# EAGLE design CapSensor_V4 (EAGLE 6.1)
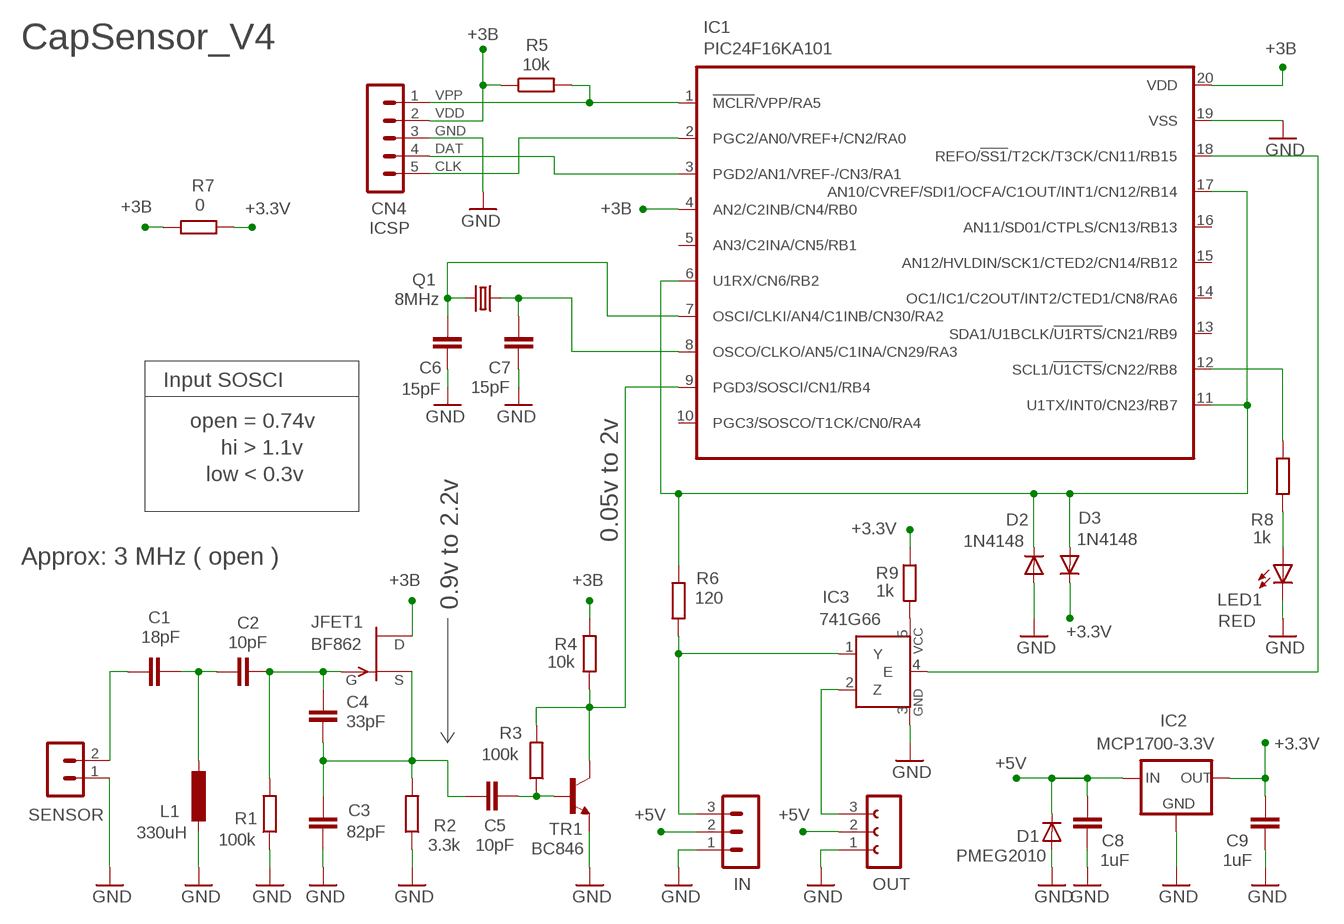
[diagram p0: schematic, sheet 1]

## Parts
C1  18pF  C-EUC0805  [C0805]
C2  10pF  C-EUC0805  [C0805]
C3  82pF  C-EUC0805  [C0805]
C4  33pF  C-EUC0805  [C0805]
C5  10pF  C-EUC0805  [C0805]
C6  15pF  C-EUC0603  [C0603]
C7  15pF  C-EUC0603  [C0603]
C8  1uF  C-EUC0603  [C0603]
C9  1uF  C-EUC0603  [C0603]
CN4  ICSP  MA05-1  [MA05-1]
D1  PMEG2010  DIODE-SOD123-B  [SOD123-B]
D2  1N4148  DIODE-SOD123-B  [SOD123-B]
D3  1N4148  DIODE-SOD123-B  [SOD123-B]
IC1  PIC24F16KA101  PIC24F04KA201SOIC  [SOIC20_S]
IC2  MCP1700-3.3V  MCP1700SOT23  [SOT23]
IC3  741G66  741G66SOT23-5L  [SOT23-5L]
IN  MA03-1N  [MA03-1]
JFET1  BF862  BF861NR  [SOT23]
L1  330uH  INDUCTORL1210  [L1210]
LED1  RED  LED3MM_F  [LED3MM]
OUT  FE03-1"  [FE03-1]
Q1  8MHz  CRYSTALC4  [CRYSTAL_4]
R1  100k  R-EU_R0805  [R0805]
R2  3.3k  R-EU_R0805  [R0805]
R3  100k  R-EU_R0805  [R0805]
R4  10k  R-EU_R0805  [R0805]
R5  10k  R-EU_R0805  [R0805]
R6  120  R-EU_R0805  [R0805]
R7  0  R-EU_R1206_L  [R1206_L]
R8  1k  R-EU_R0805_L  [R0805_L]
R9  1k  R-EU_R0603  [R0603]
SENSOR  Sensor  MA02-1N  [MA02-1]
TR1  BC846  BC846N  [SOT23]

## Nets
+3.3V: C9.1 D3.C IC2.2(OUT) R7.2 R9.1
+3B: CN4.2 IC1.4(AN2/C2INB/CN4/RB0) IC1.20(VDD) JFET1.2(D) R4.2 R5.1 R7.1
+5V: C8.1 D1.C IC2.3(IN) IN.2 OUT.2
GND: C3.1 C6.1 C7.1 C8.2 C9.2 CN4.3 D1.A D2.A IC1.19(VSS) IC2.1(GND) IC3.3(GND) IN.1 L1.2 LED1.K(C) OUT.1 R1.1 R2.1 SENSOR.1 TR1.2(E)
N$1: IC1.18(REFO/!SS1!/T2CK/T3CK/CN11/RB15) IC3.4(E)
N$2: IC1.9(PGD3/SOSCI/CN1/RB4) R3.2 R4.1 TR1.3(C)
N$3: D2.C D3.A IC1.6(U1RX/CN6/RB2) IC1.11(U1TX/INT0/CN23/RB7) IC1.17(AN10/CVREF/SDI1/OCFA/C1OUT/INT1/CN12/RB14) R6.1
N$4: C5.2 R3.1 TR1.1(B)
N$5: C1.2 C2.1 L1.1
N$6: LED1.A R8.2
N$7: C3.2 C4.1 C5.1 JFET1.1(S) R2.2
N$8: IC1.12(SCL1/!U1CTS!/CN22/RB8) R8.1
N$9: C2.2 C4.2 JFET1.3(G) R1.2
N$10: C1.1 SENSOR.2
N$11: IC3.5(VCC) R9.2
N$13: C6.2 IC1.7(OSCI/CLKI/AN4/C1INB/CN30/RA2) Q1.3
N$14: C7.2 IC1.8(OSCO/CLKO/AN5/C1INA/CN29/RA3) Q1.1
N$15: IC3.2(Z) OUT.3
N$16: IC3.1(Y) IN.3 R6.2
N$18: CN4.4 IC1.3(PGD2/AN1/VREF-/CN3/RA1)
N$19: CN4.1 IC1.1(!MCLR!/VPP/RA5) R5.2
N$20: CN4.5 IC1.2(PGC2/AN0/VREF+/CN2/RA0)
Unconnected: IC1.5(AN3/C2INA/CN5/RB1) IC1.10(PGC3/SOSCO/T1CK/CN0/RA4) IC1.13(SDA1/U1BCLK/!U1RTS!/CN21/RB9) IC1.14(OC1/IC1/C2OUT/INT2/CTED1/CN8/RA6) IC1.15(AN12/HVLDIN/SCK1/CTED2/CN14/RB12) IC1.16(AN11/SD01/CTPLS/CN13/RB13)

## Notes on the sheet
- CapSensor_V4
- Input SOSCI
- open = 0.74v
- hi > 1.1v
- low < 0.3v
- 0.05v to 2v
- Approx: 3 MHz ( open )
- 0.9v to 2.2v

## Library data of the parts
C1-C9 = 00-LIVIO:C-EU: CAPACITOR, European symbol
CN4 = 03-con-lstb-M:MA05-1: PIN HEADER; CLK: CLK; DAT: DAT; GND: GND; VDD: VDD; VPP: VPP
D1-D3 = 00-LIVIO:DIODE-: DIODE
IC1 = 00-LIVIO:PIC24F04KA201
IC2 = 00-LIVIO:MCP1700: Linear regulator Quescient courrent 1.8uA Input 2.3v to 6v Output 1.2v 1.8v 2.5v 3.0v 3.3v 5.0v
IC3 = 00-LIVIO:74*1G66: Single Analog / Bilateral Switch Source: http://www.semiconductors.philips.com/acrobat_download/datasheets/74HC_HCT1G66_3.pdf
IN = 03-con-lstb-M:MA03-1: PIN HEADER
JFET1 = 00-LIVIO:BF861
L1 = 00-LIVIO:INDUCTOR
LED1 = 00-LIVIO:LED: LEDS
OUT = 02-con-lsta-F:FE03-1: FEMALE HEADER
Q1 = 00-LIVIO:CRYSTAL: CRYSTAL
R1-R9 = 00-LIVIO:R-EU_: RESISTOR, European symbol
SENSOR = 03-con-lstb-M:MA02-1: PIN HEADER
TR1 = 00-LIVIO:BC846

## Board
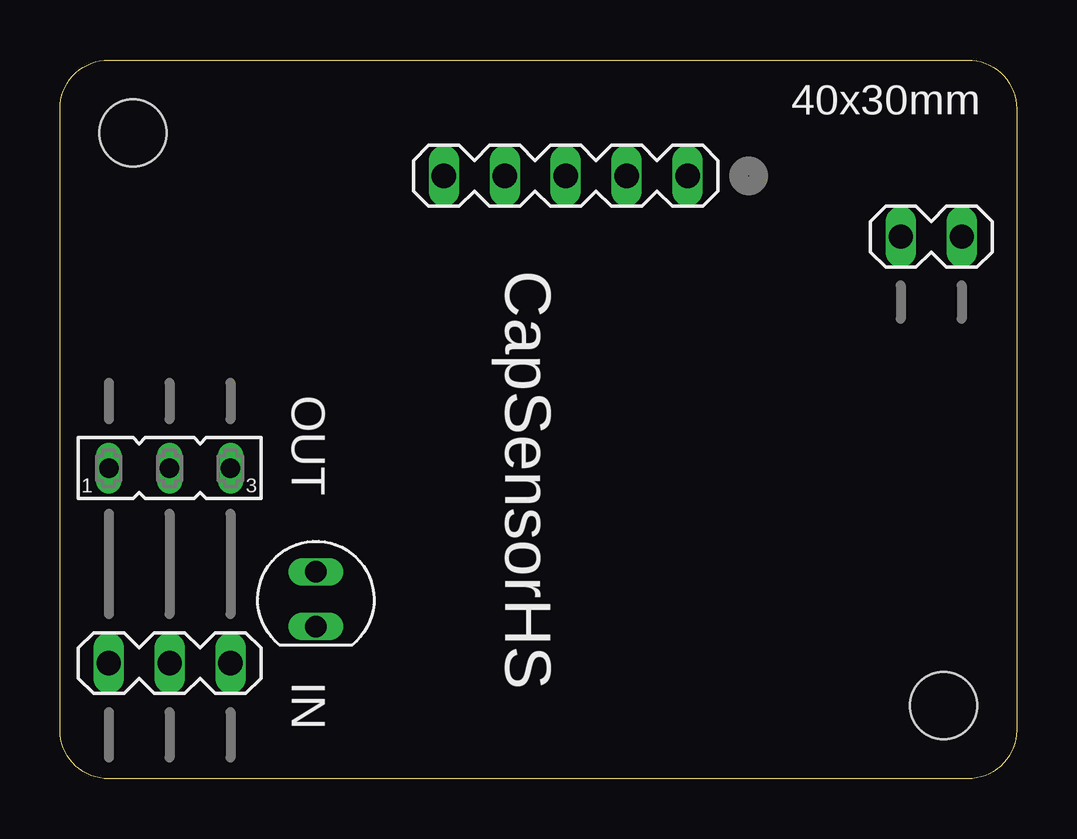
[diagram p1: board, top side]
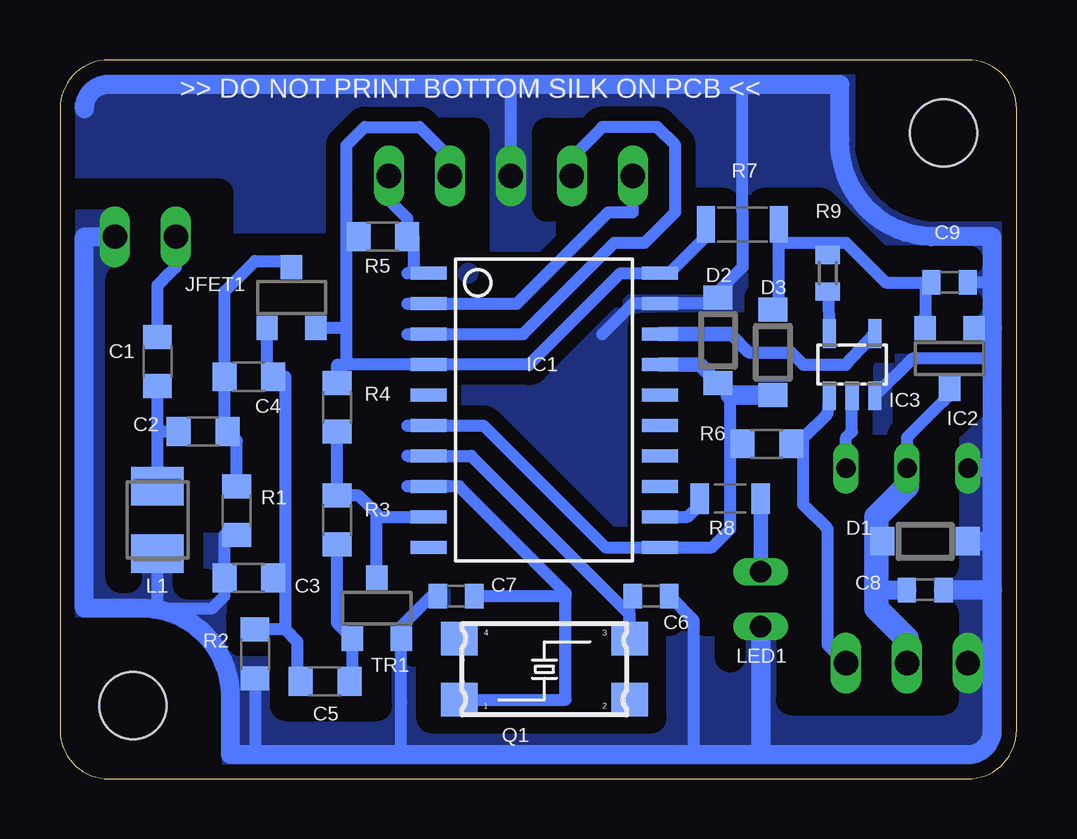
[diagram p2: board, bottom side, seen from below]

Size 39.88 x 29.97 mm. Coordinates in mm from the lower left corner, seen from the top.
Outline: 37.85,0 2.03,0 arc-90 0,2.03 0,27.94 arc-90 2.03,29.97 37.85,29.97 arc-90 39.88,27.94 39.88,2.03 arc-90 37.85,0
Copper layers (1*16): Top 0.035mm / dielectric 1.5mm / Bottom 0.035mm
Design rules: minimum track width 10mil, minimum drill 19mil, track to track 19mil, track to pad 19mil, pad to pad 19mil, via to via 19mil, smd to smd 19mil, copper to edge 19mil, drill to drill 8mil, minimum pad ring 5mil, minimum via ring 8mil, stop-mask expansion 4mil, vias tented up to drill 0mil, thermal gap 29mil
Holes 2.8 mm at 3.05,26.92 36.83,3.05
bRestrict: area 4.3,15.5 to 4.6,16.5; 58 lines

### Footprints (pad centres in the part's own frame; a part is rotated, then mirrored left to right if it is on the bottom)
C0805 = smd 1 x 1.2: 1 -1.016,0; 2 1.016,0
C0603 = smd 0.762 x 1.016: 1 -0.762,0; 2 0.762,0
MA05-1 = drill 1.016 long: 1 -5.08,0; 2 -2.54,0; 3 0,0; 4 2.54,0; 5 5.08,0
SOD123-B = smd 1 x 1.2: A 1.778,0; C -1.778,0
SOIC20_S = smd 0.55 x 1.5: 1 -5.715,-4.826; 2 -4.445,-4.826; 3 -3.175,-4.826; 4 -1.905,-4.826; 5 -0.635,-4.826; 6 0.635,-4.826; 7 1.905,-4.826; 8 3.175,-4.826; 9 4.445,-4.826; 10 5.715,-4.826; 11 5.715,4.826; 12 4.445,4.826; 13 3.175,4.826; 14 1.905,4.826; 15 0.635,4.826; 16 -0.635,4.826; 17 -1.905,4.826; 18 -3.175,4.826; 19 -4.445,4.826; 20 -5.715,4.826
SOT23 = smd 0.889 x 1.016: 1 -1.016,-1.27; 2 1.016,-1.27; 3 0,1.27
SOT23-5L = smd 0.55 x 1.2: 1 -0.95,-1.3; 2 0,-1.3; 3 0.95,-1.3; 4 0.95,1.3; 5 -0.95,1.3
MA03-1 = drill 1.016 long: 1 -2.54,0; 2 0,0; 3 2.54,0
L1210 = smd 1.6 x 2.2: 1 -1.4,0; 2 1.4,0
LED3MM = drill 0.9 long: A -1.016,0; K 1.27,0
FE03-1 = drill 0.813 long: 1 -2.54,0; 2 0,0; 3 2.54,0
CRYSTAL_4 = smd 1.524 x 1.397: 1 -3.556,-1.27; 2 3.556,-1.27; 3 3.556,1.27; 4 -3.556,1.27
R0805 = smd 1 x 1.2: 1 -1.016,0; 2 1.016,0
R1206_L = smd 0.762 x 1.524: 1 -1.524,0; 2 1.524,0
R0805_L = smd 0.762 x 1.27: 1 -1.27,0; 2 1.27,0
R0603 = smd 0.762 x 1.016: 1 -0.762,0; 2 0.762,0
MA02-1 = drill 1.016 long: 1 -1.27,0; 2 1.27,0

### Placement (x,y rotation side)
C1  35.81,17.4 270 bottom
C2  33.91,14.48 0 bottom
C3  32,8.38 0 bottom
C4  32,16.76 180 bottom
C5  28.83,4.06 0 bottom
C6  15.24,7.62 180 bottom
C7  23.37,7.62 0 bottom
C8  3.81,7.87 0 bottom
C9  2.79,20.7 0 bottom
CN4  21.08,25.15 180 top
D1  3.81,9.91 0 bottom
D2  12.45,18.29 90 bottom
D3  10.16,17.78 270 bottom
IC1  19.68,15.37 270 bottom
IC2  2.79,17.53 180 bottom
IC3  6.86,17.27 0 bottom
IN  4.57,4.83 0 top
JFET1  30.23,20.07 0 bottom
L1  35.81,10.79 270 bottom
LED1  10.67,7.62 270 top
OUT  4.57,12.95 0 top
Q1  19.68,4.57 0 bottom
R1  32.51,11.18 90 bottom
R2  31.75,5.21 90 bottom
R3  28.32,10.79 90 bottom
R4  28.32,15.49 90 bottom
R5  26.42,22.61 0 bottom
R6  10.41,13.97 0 bottom
R7  11.43,23.11 0 bottom
R8  11.94,11.68 0 bottom
R9  7.87,21.08 270 bottom
SENSOR  36.32,22.61 180 top
TR1  26.67,7.11 0 bottom

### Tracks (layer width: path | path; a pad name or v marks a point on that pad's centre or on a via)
+3.3V
  Bottom 0.508: IC2.2 3.81,19.3 3.81,20.7 | 9.91,22.35 7.87,22.35 | 7.87,22.35 7.11,22.35 5.46,20.7 3.81,20.7 | 3.81,20.7 C9.1 3.81,20.7 | 9.91,22.35 9.91,19.56 D3.C | R9.1 7.87,22.35 | 9.91,22.35 R7.2
+3B
  Bottom 0.508: 27.94,18.8 JFET1.2 | 27.94,17.27 27.94,18.8 | 27.94,22.61 27.94,23.37 27.94,23.88 27.94,26.42 27.18,27.18 24.89,27.18 23.62,25.91 CN4.2 | 27.94,18.8 27.94,22.61 | 27.94,17.27 28.32,17.27 R4.2 | 27.94,17.27 IC1.4 20.32,17.27 16.51,21.08 IC1.20 14.48,21.08 12.95,22.61 R7.1 | R5.1 27.94,22.61
+5V
  Bottom 0.508: IC2.3 2.79,16 3.05,15.75 4.57,14.22 OUT.2 4.57,12.45 4.57,12.19 | IN.2 4.57,5.59 4.57,5.84
  Bottom 0.8: 5.84,7.87 C8.1 5.84,7.87
  Bottom 1.016: 4.57,5.84 5.84,7.11 5.84,7.87 5.84,9.91 | 5.84,9.91 D1.C 5.84,9.91 | 5.84,9.91 5.84,10.92 4.57,12.19
GND
  Bottom 0.508: R1.1 33.02,10.16 C3.1 33.02,8.13 33.02,7.62 33.27,7.37 33.53,7.11 35.81,7.11 | 38.86,7.11 36.32,7.11 35.81,7.11 | 35.81,7.11 L1.2 | 25.65,1.02 25.65,3.21 TR1.2 25.65,6.35 24.38,7.62 C7.1 | IC3.3 4.32,17.53 1.02,17.53 | 1.02,20.7 C9.2 | 17.27,18.54 16,19.81 IC1.19 12.7,19.81 D2.A 12.45,20.32 11.43,21.34 11.43,23.62 11.43,28.96 | CN4.3 21.08,28.96 | R2.1 31.75,1.02 | C6.1 13.46,6.6 13.46,1.02
  Bottom 0.8: 1.02,4.83 1.02,2.03 arc90 2.03,1.02 10.67,1.02 13.46,1.02 25.65,1.02 31.75,1.02 32.77,1.02 32.77,3.3 arc-90 36.32,7.11 38.86,7.11 38.86,22.61 SENSOR.1 | 1.02,4.83 IN.1 | 1.02,4.83 1.02,7.62 1.02,7.87 | 1.02,9.91 D1.A | 1.02,7.87 1.02,9.91 | 1.02,9.91 1.02,12.95 | 1.02,12.95 1.02,17.53 1.02,18.8 1.02,20.7 1.02,22.61 3.56,22.61 arc90 7.37,26.67 7.37,28.96 11.43,28.96 21.08,28.96 37.85,28.96 arc-90 38.86,27.94 | C8.2 1.02,7.87 | 1.02,12.95 OUT.1
  Bottom 0.813: 1.02,18.8 IC2.1 | 10.67,1.02 LED1.K | 1.02,7.87 C8.2
  pour Bottom (isolate 0.6, no thermals): -1,-1 40.88,-1 40.88,30.97 -1,30.97
N$1
  Bottom 0.508: IC3.4 7.11,17.27 8.89,17.27 9.4,17.78 11.18,17.78 11.94,18.54
  Bottom 0.61: IC1.18 11.94,18.54
N$2
  Bottom 0.508: 26.67,10.92 26.54,10.92 | 26.54,10.92 27.43,11.81 R3.2 R4.1 | 26.67,10.92 26.54,10.92 | 26.54,10.92 IC1.9 | TR1.3 26.67,10.92
N$3
  Bottom 0.508: 11.94,13.97 11.94,10.41 12.7,9.65 IC1.11 17.14,9.65 22.23,14.73 IC1.6 25.4,14.73 | 11.94,13.97 R6.1 | 11.94,13.97 11.94,16
  Bottom 0.61: 11.94,16 D2.C 13.21,17.27 IC1.17
  Bottom 0.813: 11.94,16 D3.A
N$4
  Bottom 0.508: R3.1 28.32,6.48 TR1.1 27.69,4.06 C5.2
N$5
  Bottom 0.508: L1.1 35.81,14.48 | 35.81,14.48 C2.1 | 35.81,14.48 C1.2
N$6
  Bottom 0.61: LED1.A R8.2
N$7
  Bottom 0.508: 30.48,8.38 30.48,15.24 30.48,16.76 C4.1 31.24,16.76 JFET1.1 | 30.48,8.38 C3.2 | C5.1 29.97,4.06 29.97,5.71 30.48,6.22 | 30.48,6.22 30.48,8.38 | 30.48,6.22 R2.2
N$8
  Bottom 0.508: R8.1 13.21,11.43 13.72,10.92 IC1.12
N$9
  Bottom 0.508: JFET1.3 30.23,21.59 31.75,21.59 33.02,20.32 C4.2 33.02,14.61 C2.2 32.51,14.1 R1.2
N$10
  Bottom 0.508: C1.1 35.81,20.57 35.31,21.08 35.05,21.34 SENSOR.2
N$11
  Bottom 0.508: R9.2 IC3.5
N$12
  pour Bottom (no thermals): 22.48,21.08 arc180 23.24,21.08 arc180
N$13
  Bottom 0.508: C6.2 16.13,7.62 Q1.3 16.13,6.86 22.73,13.46 IC1.7 25.4,13.46
N$14
  Bottom 0.508: 18.8,7.75 23.24,12.19 IC1.8 25.4,12.19 | Q1.1 18.8,3.3 18.8,7.62 | 18.8,7.62 18.8,7.75 | C7.2 18.8,7.62 | 18.8,7.75 18.8,7.62
N$15
  Bottom 0.508: IC3.2 6.86,14.48 7.11,14.22 OUT.3
N$16
  Bottom 0.508: 8.89,13.97 8.89,14.22 7.87,15.24 IC3.1 | IN.3 7.87,5.59 7.87,10.41 8.89,11.43 8.89,13.97 | 8.89,13.97 R6.2
N$18
  Bottom 0.508: 25.4,18.54 IC1.3 20.57,18.54 16.76,22.35 15.49,22.35 14.22,23.62 14.22,26.42 14.99,27.18 17.27,27.18 18.54,25.91 CN4.4
N$19
  Bottom 0.305: 25.15,21.08 IC1.1
  Bottom 0.508: IC1.1 25.15,21.08 | 25.15,21.08 25.4,21.08 | 25.15,21.08 25.15,22.61 R5.2 25.4,23.37 26.16,24.13 CN4.1
N$20
  Bottom 0.508: 25.4,19.81 IC1.2 20.83,19.81 17.02,23.62 16,23.62 CN4.5

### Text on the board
tNames: 40x30mm | CapSensorHS
bNames: >> DO NOT PRINT BOTTOM SILK ON PCB <<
